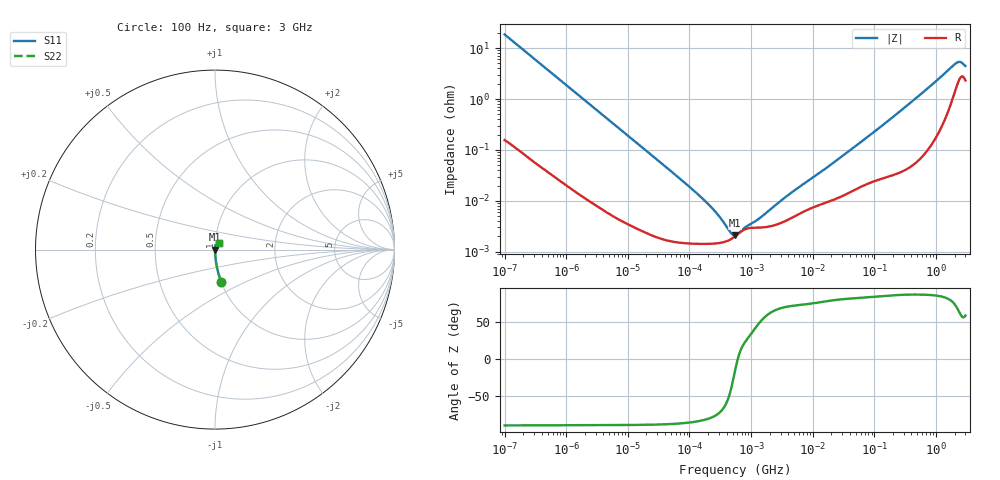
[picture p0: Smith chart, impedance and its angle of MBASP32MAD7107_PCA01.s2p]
! MBASP32MAD7107_PCA01  S-PARAMETER MODEL  ( Standard Model )
! Model Generated by TAIYO YUDEN Corporation (http://www.ty-top.com)
! Version 1.0
! TAIYO YUDEN Control No. 241206
! Copyright(c) 2024 TAIYO YUDEN CO.,LTD. All Rights Reserved.
! Product Description (link to TY-COMPAS)
! https://ds.yuden.co.jp/TYCOMPAS/or/detail?pn=MBASP32MAD7107MPCA01&u=M
! Products Name : Multilayer Ceramic Capacitors
! Characteristics :
!  Capacitance : 100 [uF] , Rated Voltage : 2.5 [V] , TCC : X7T
!  Case Size : 3.2 x 2.5 / 0.126 x 0.098 [mm/inch] , Thickness : 2.5 / 0.098 [mm/inch]
!  (Conditions: Temperature = 25 [degC] , DC Bias Voltage = 0 [V])
! External Node Assignments :
!  1  o---| |---o  2
! GND o---------o GND
! Frequency Range : 100Hz  -  3GHz  [ 401 STEP ]
# MHZ S RI R 50
! Freq[MHz].  S11 Real  S11 Imag  S21 Real  S21 Imag  S12 Real  S12 Imag  S22 Real  S22 Imag
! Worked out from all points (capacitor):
!   401 points, 100 Hz to 3 GHz, reference 50 ohm
!   read as one part in series: C = 85.9 uF near 109 Hz
!   lowest |Z| = 2.09 mohm at 547.7 kHz (marker M1)
!   series resonance near 607.6 kHz, so ESL is about 800 pH
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0.0001  0.0345 -0.1783  0.9655 0.1783  0.9655 0.1783  0.0345 -0.1783
0.000114  0.0271 -0.1581  0.9729 0.1581  0.9729 0.1581  0.0271 -0.1581
0.000175  0.0121 -0.1047  0.9879 0.1047  0.9879 0.1047  0.0121 -0.1047
0.000306  0.00425 -0.0605  0.9958 0.0605  0.9958 0.0605  0.00425 -0.0605
0.000664  0.00108 -0.0281  0.9989 0.0281  0.9989 0.0281  0.00108 -0.0281
0.001788  0.000234 -0.0105  0.9998 0.0105  0.9998 0.0105  0.000234 -0.0105
0.031977  1.89e-05 -0.0006  1 0.0006  1 0.0006  1.89e-05 -0.0006
0.089839  1.47e-05 -0.00021  1 0.00021  1 0.00021  1.47e-05 -0.00021
0.16412  1.43e-05 -0.000109  1 0.000109  1 0.000109  1.43e-05 -0.000109
0.178874  1.43e-05 -9.87e-05  1 9.87e-05  1 9.87e-05  1.43e-05 -9.87e-05
0.194955  1.43e-05 -8.89e-05  1 8.89e-05  1 8.89e-05  1.43e-05 -8.89e-05
0.547723  2.01e-05 -5.79e-06  1 5.79e-06  1 5.79e-06  2.01e-05 -5.79e-06
2.93481  3.61e-05 9.02e-05  1 -9.02e-05  1 -9.02e-05  3.61e-05 9.02e-05
3.339322  3.85e-05 0.000103  1 -0.000103  1 -0.000103  3.85e-05 0.000103
9.794414  7.32e-05 0.000271  0.9999 -0.000271  0.9999 -0.000271  7.32e-05 0.000271
25.2476  0.000113 0.000633  0.9999 -0.000633  0.9999 -0.000633  0.000113 0.000633
175.1444  0.000318 0.00388  0.9997 -0.00388  0.9997 -0.00388  0.000318 0.00388
694.33  0.00114 0.0153  0.9989 -0.0153  0.9989 -0.0153  0.00114 0.0153
2036.508  0.016 0.0452  0.984 -0.0452  0.984 -0.0452  0.016 0.0452
2219.584  0.0212 0.0466  0.9788 -0.0466  0.9788 -0.0466  0.0212 0.0466
2419.119  0.0264 0.0451  0.9736 -0.0451  0.9736 -0.0451  0.0264 0.0451
3000  0.024 0.0362  0.976 -0.0362  0.976 -0.0362  0.024 0.0362
